ORGANIZATION_BLOCK MAIN:OB1
TITLE= Miscelatore di due liquidi
// Simulatore: 12
// Versione: 1.0
// Data: 24/01/2002
// Il processo di miscelazione e scarico del prodotto avviene
// completamente in automatico.
// Il ciclo viene avviato agendo sul pulsante di start (SB11)
// e può essere interrotto in qualsiasi momento dal pulsante
// di Stop (SB10). Dopo un arresto, al successivo riavvio,
// il ciclo riprenderà dalla fase in cui era stato interrotto,
// e la fase stessa verrà completata prima di passare alla
// successiva.
// Due contatori software (C1 e C2) provvedono a contare gli
// impulsi forniti dai traduttori di flusso (TF1, TF2) e
// quindi a contare i litri di prodotto che transitano nelle
// rispettive tubazioni verso il serbatoio.
// Ogni contatore sarà preimpostato sui litri di prodotto da
// caricare nel serbatoio (C1=60, C2=100) tenendo presente che
// la capacità massima (virtuale) del sebatoio è di 160 litri.
// Le fasi del processo sono così suddivise:
// 1) Carico della quantità impostata dei due prodotti
//    operata dall'apertura delle elettrovalvole  (YV1, YV2)
//    e dalla messa in funzione delle pompe (P1, P2)
// 2) Quando il carico è completato inizia una fase di
//    riscaldamento (apertura dell'elettrovalvola YV4 che
//    immette vapore nel serbatoio) e mescolazione (motore M3
//    che aziona un mescolatore). La durata di questa fase è
//    gestita dal temporizzatore T32.
// 3) Trascorso il tempo della fase precedente viene
//    avviato lo scarico del prodotto (elettrovalvola YV3)
//    e quando il serbatoio si è completamente svuotato
//    riprende un nuovo ciclo.
// Le informazione sul livello (Minimo, Massimo) del serbatoio
// vengono ricavate dai due bit (TL1,TL2) del trasduttore
// di livello e vengono memorizzate in due marker
// M1.0 (Minimo) e M1.1 (Massimo), il marker M0.1 memorizzerà
// la condizione di carico dei prodotti completata (che può
// non corrispondere alla condizione di serbatoio pieno).
// Quattro lampade segnalono rispettivamente:
//   HL1: Pompa P1 in funzione
//   HL2: Pompa P2 in funzione
//   HL3: Fase di riscaldamento e miscelazione
//   HL4: Fase di scarico
//

BEGIN
NETWORK 1
LD SM0.1
R M0.0 7
R M1.0 7
R M2.0 7
R M3.0 7
R M4.0 7

NETWORK 2 //Carica Tempo riscaldamento da potenziometro analogico
//
LD SM0.0
MOVB SMB28 AC0

NETWORK 3 //Se valore caricato =0n imposta  valore 50
//
LD SM0.0
AB= AC0 0
MOVB 50 AC0

NETWORK 4 //Impostazione per funzionamento automatico/Manuale
//
LD I0.5
= S0.0
NOT
= S0.1

NETWORK 5 //Imposta Merker  Serbatoio Pieno
//
LD I0.2
A I0.3
= M1.1

NETWORK 6 //Imposta Merker Serbatoio Vuoto
//
LDN I0.2
AN I0.3
= M1.0

NETWORK 7 //Inizio blocco controllo manuale
//
LSCR S0.1

NETWORK 8 //Mandata prodotto 1
//
LD I1.0
O M4.0
A I1.1
AN M1.1
= M4.0

NETWORK 9 //Mandata prodotto 2
//
LD I1.2
O M4.1
A I1.3
AN M1.1
= M4.1

NETWORK 10 //Comando miscelatore e riscaldatore
//
LD I1.4
O M4.2
A I1.5
AN Q0.4
AN M1.0
= M4.2

NETWORK 11 //Comando Scarico Miscela
//
LD I1.6
O M4.3
A I1.7
AN M1.0
= M4.3

NETWORK 12 //Fine blocco controllo manuale
//
SCRE

NETWORK 13 //Inizio blocco controllo automatico
//
LSCR S0.0

NETWORK 14 //Contatore prodotto 1
//
LD I0.0
LD M1.0
CTU C0 +20

NETWORK 15 //Contatore prodotto 2
//
LD I0.1
LD M1.0
CTU C1 +30

NETWORK 16 //Carico miscela completato
//
LD C1
A C0
= M0.1

NETWORK 17 //Gestione ciclo automatico
//
LD I0.6
A M1.0
O M0.2
A I0.7
AN M1.1
= M0.2

NETWORK 18 //Gestione carico prodotto 1
//
LD M0.2
AN C0
= M3.0

NETWORK 19 //Gestione carico prodotto 2
//
LD M0.2
AN C1
= M3.1

NETWORK 20 //Gestione Micelazione/Riscaldamento
//
LD M0.1
AN T32
= M3.2

NETWORK 21 //Temporizzatore fase riscaldamento
//
LD M0.1
TON T32 AC0

NETWORK 22 //Gestione scarico miscela
//
LD T32
AN M1.0
= M3.3

NETWORK 23 //Segnalazione errore di caricamento
//
LD M1.1
LDN C0
ON C1
ALD
= Q1.5

NETWORK 24 //Fine blocco controllo automatico
//
SCRE

NETWORK 25 //Comando uscite carico prodotto 1
//
LD M3.0
O M4.0
= Q0.1
= Q0.0
= Q0.6

NETWORK 26 //Comando uscite carico prodotto 2
//
LD M3.1
O M4.1
= Q0.2
= Q0.3
= Q0.7

NETWORK 27 //Comando uscite Miscelazione e Vapore
//
LD M3.2
O M4.2
= Q0.5
= Q1.6
= Q1.0

NETWORK 28 //Comando uscita valvola di scarico
//
LD M3.3
O M4.3
= Q0.4
= Q1.1

NETWORK 29 //Segnalazione modo Manuale
//
LD S0.1
= Q1.2

NETWORK 30 //Segnalazione modo Automatico
//
LD S0.0
A SM0.5
O M0.2
= Q1.3

END_ORGANIZATION_BLOCK

